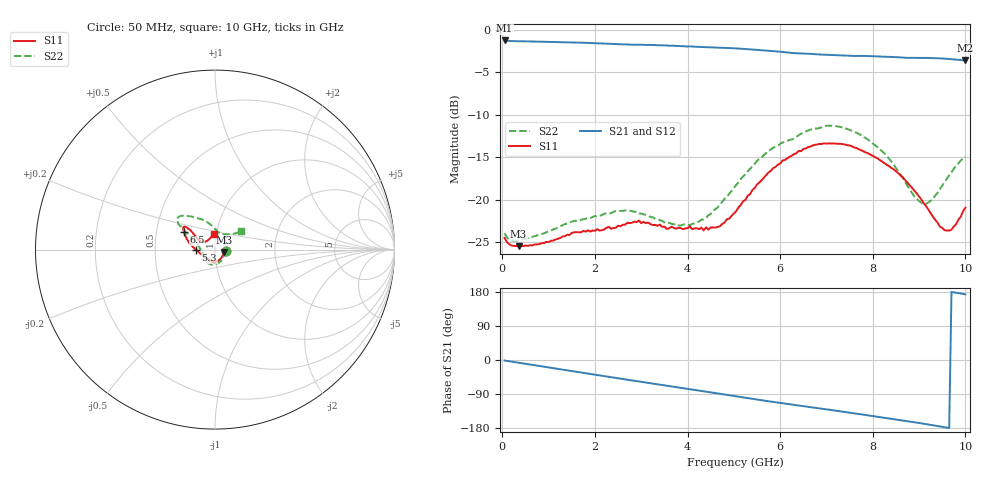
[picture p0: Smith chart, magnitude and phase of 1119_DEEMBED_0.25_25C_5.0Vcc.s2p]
!Hittite Microwave Corp.
!Digital Attenuator/PhaseShifter Rev 1.4.0
!Filename: C:\DATA\DATA\1119_DEEMBED_0.25_25C_5.0Vcc.s2p
!VNA ID: Agilent Technologies,N5224A,MY51441122,A.10.45.03
!Device type:
!2 Port Calibration.
!Temp(C): 25
!Lot Number:
!Serial Number:
!Operator:
!Misc:
!Attenuator:  0.250
# GHZ S DB R 50.0
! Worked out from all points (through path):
!   200 points, 50 MHz to 10 GHz, reference 50 ohm
!   highest |S21| = -1.24 dB at 50 MHz (marker M1); lowest = -3.6 dB at 10 GHz (marker M2)
!   group delay of S21, straight-line fit = 51 ps
!   lowest |S11| = -25.5 dB at 350 MHz (marker M3), VSWR 1.11, Z = 55.3 - j1.75 ohm
!   |S11| at or under -10 dB: start of sweep to end of sweep
!   |S22| runs from -24.8 to -11.3 dB; largest |S21 - S12| = 0.0021
!   S11 on the Smith chart (normalised r, x): 50 MHz: 1.12, -0.02; 5.3 GHz: 0.81, -0.00; 6.5 GHz: 0.69, +0.14; 10 GHz: 0.97, +0.17
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0.05  -24.53 -8.4  -1.24 -1.5  -1.24 -1.4  -23.97 -8.4
0.35  -25.50 -17.3  -1.33 -7.2  -1.33 -7.2  -24.80 -18.7
1.75  -23.69 -74.4  -1.51 -34.1  -1.51 -34.1  -22.31 -76.1
2.65  -22.97 -88.0  -1.72 -51.0  -1.71 -51.1  -21.28 -108.4
2.95  -22.48 -93.4  -1.74 -56.4  -1.75 -56.5  -21.63 -119.8
3.4  -22.96 -100.8  -1.80 -64.9  -1.80 -65.0  -22.42 -134.7
3.85  -23.37 -107.5  -1.91 -73.4  -1.91 -73.5  -23.07 -150.0
4.35  -23.64 -122.6  -2.02 -82.6  -2.03 -82.7  -22.35 -176.3
4.7  -23.14 -142.8  -2.10 -89.1  -2.12 -89.2  -20.61 167.2
5.05  -21.38 -165.3  -2.18 -95.7  -2.19 -95.8  -18.29 156.6
5.3  -19.56 -178.7  -2.26 -100.5  -2.27 -100.5  -16.70 153.4
5.85  -16.29 163.8  -2.50 -110.8  -2.51 -110.9  -13.88 147.8
6.5  -14.05 150.9  -2.78 -121.7  -2.79 -121.8  -12.10 144.9
6.7  -13.63 148.1  -2.84 -125.2  -2.85 -125.3  -11.69 142.8
7.45  -13.59 142.8  -3.03 -138.1  -3.03 -138.2  -11.68 133.5
8.35  -16.06 142.8  -3.16 -154.4  -3.16 -154.4  -15.17 110.6
8.9  -18.97 148.5  -3.29 -164.3  -3.29 -164.3  -19.63 84.1
9.15  -20.78 150.3  -3.29 -169.2  -3.30 -169.2  -20.50 67.4
9.45  -23.21 141.5  -3.35 -175.3  -3.36 -175.3  -18.79 47.5
9.6  -23.66 129.1  -3.41 -178.4  -3.42 -178.4  -17.53 41.1
9.799999  -22.91 108.3  -3.49 177.4  -3.50 177.4  -16.02 36.8
10  -20.97 93.9  -3.59 173.3  -3.60 173.3  -14.93 35.3
